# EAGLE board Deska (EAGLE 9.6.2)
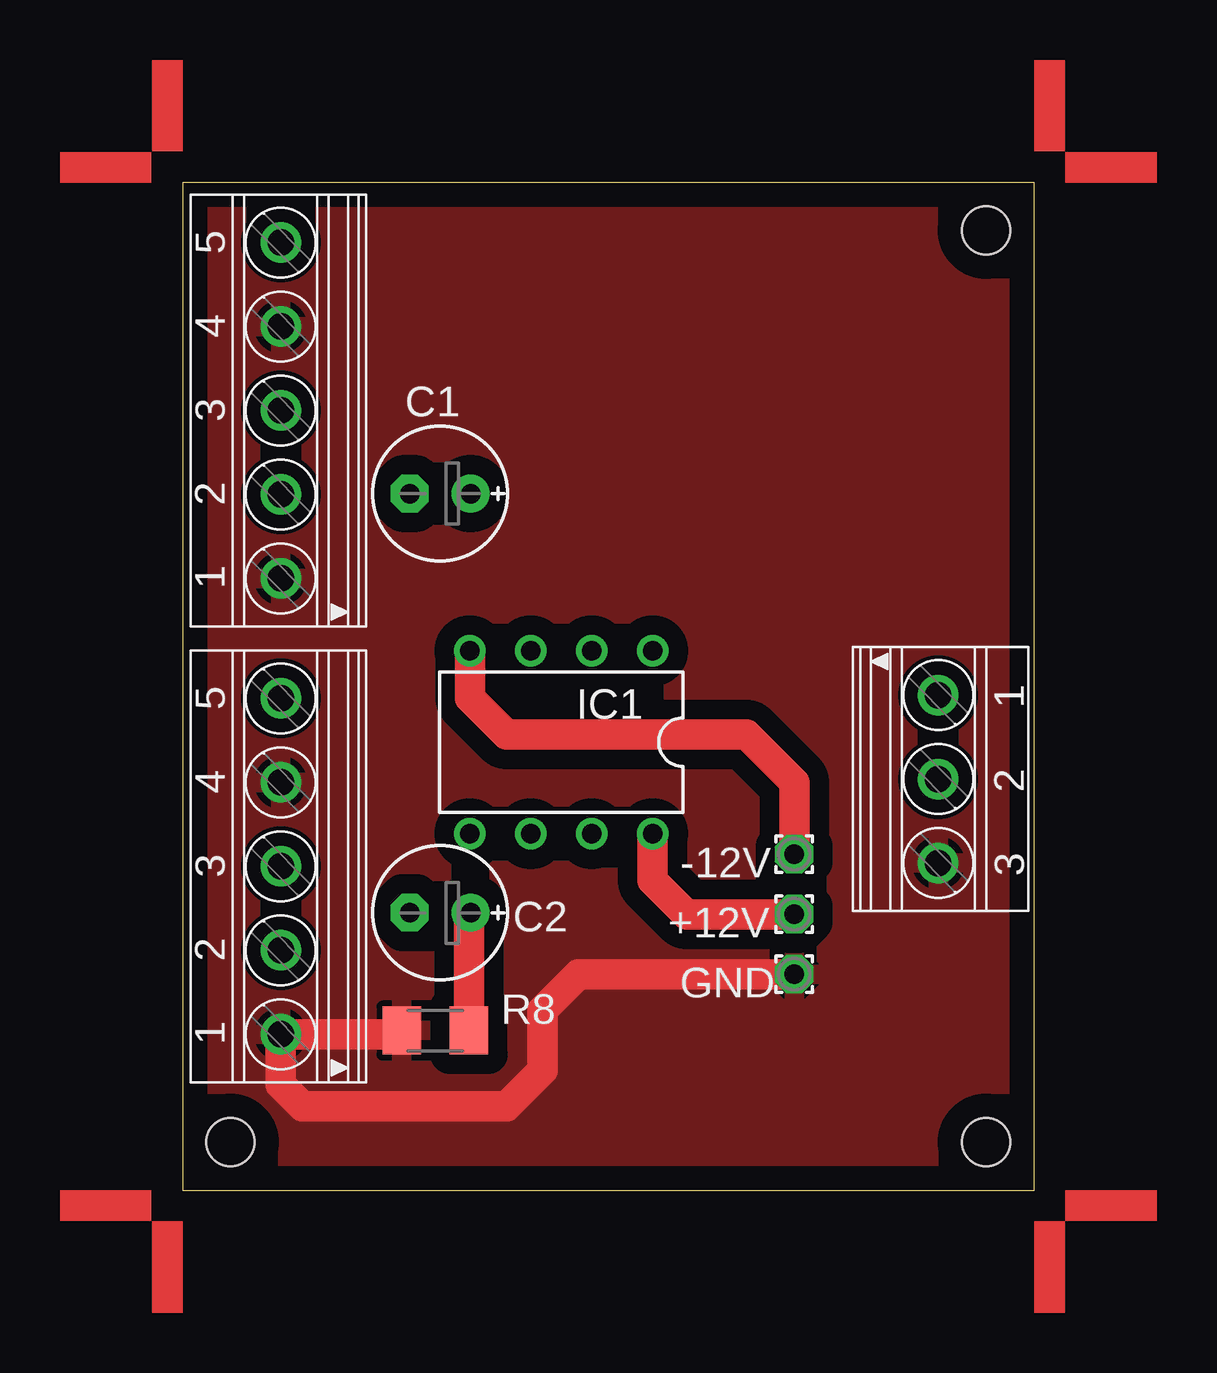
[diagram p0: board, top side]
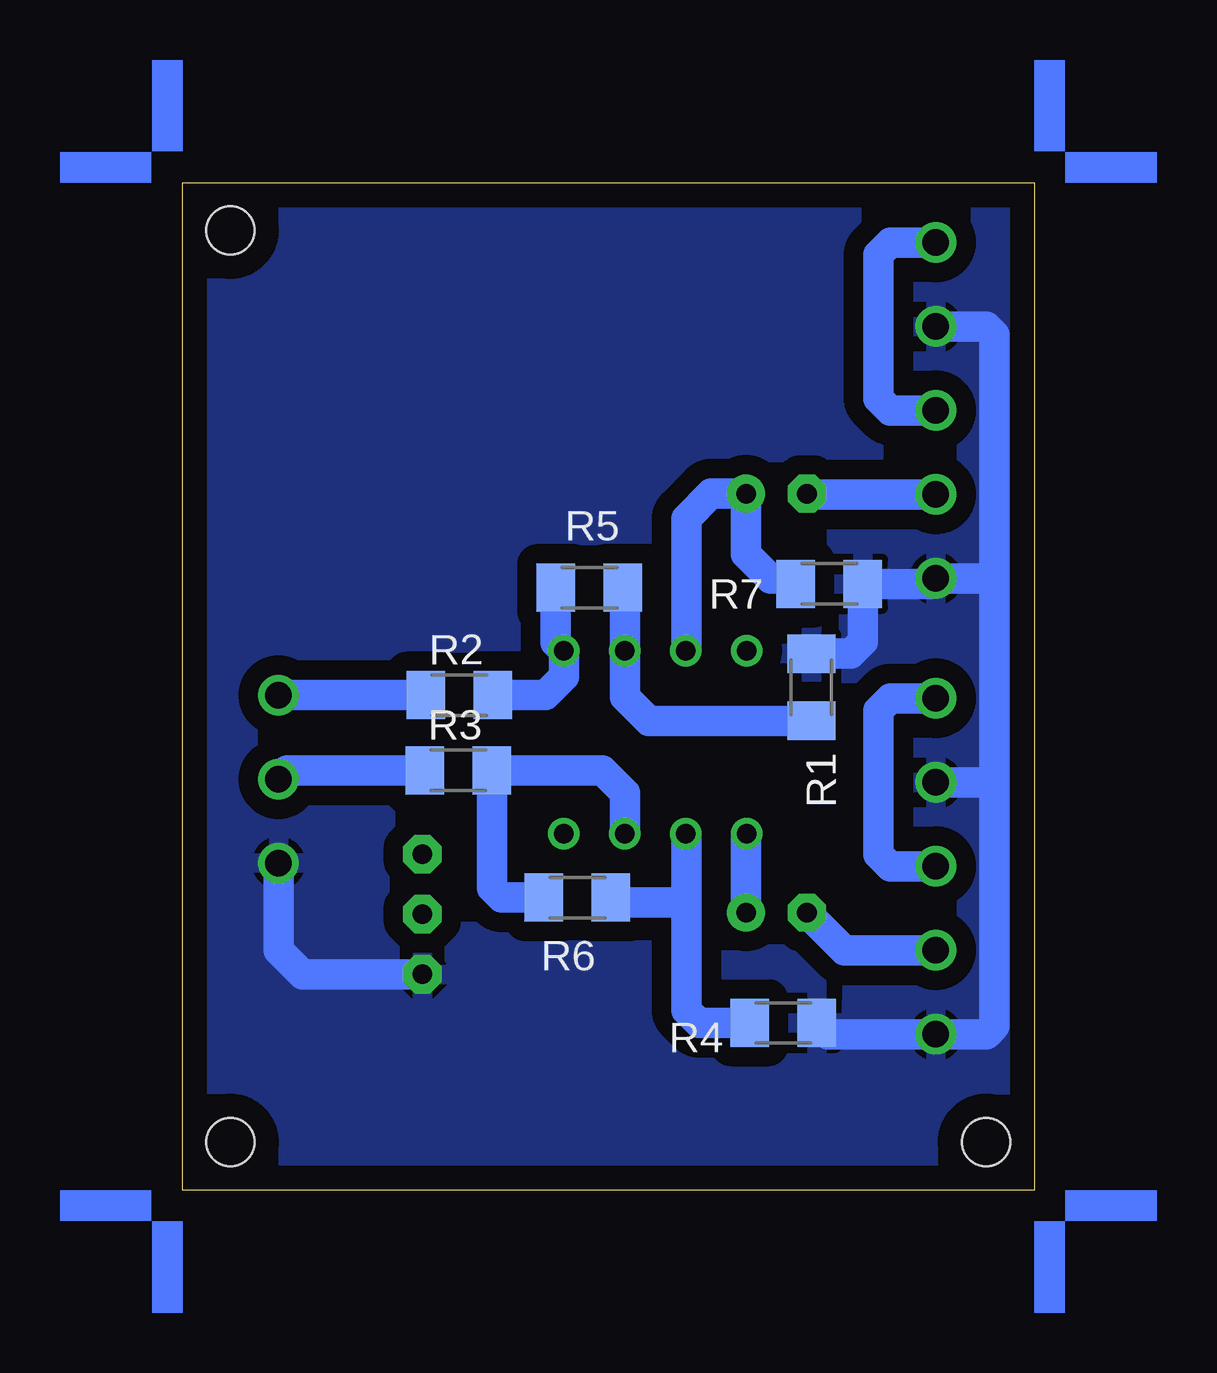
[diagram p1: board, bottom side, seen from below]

Size 35.5 x 42 mm. Coordinates in mm from the lower left corner, seen from the top.
Outline: 0,0 35.5,0 35.5,42 0,42 0,0
Copper layers (1*16): Top 0.035mm / dielectric 1.5mm / Bottom 0.035mm
Design rules "default": minimum track width 6mil, minimum drill 0.35mm, track to track 6mil, track to pad 6mil, pad to pad 6mil, via to via 6mil, smd to smd 6mil, copper to edge 40mil, drill to drill 6mil, minimum pad ring 10mil, minimum via ring 8mil, stop-mask expansion 4mil, vias tented up to drill 0mil, thermal gap 10mil
Holes 2 mm at 2,2 33.5,2 33.5,40

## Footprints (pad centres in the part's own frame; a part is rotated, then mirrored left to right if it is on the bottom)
1,6/0,8 = drill 0.813 pad 1.6 octagon: 1 0,0
E2,5-6E = drill 0.813 pad 1.575: + -1.27,0 | drill 0.813 pad 1.575 octagon: - 1.27,0
DIL08 = drill 0.813 pad 1.27: 1 -3.81,-3.81; 2 -1.27,-3.81; 3 1.27,-3.81; 4 3.81,-3.81; 5 3.81,3.81; 6 1.27,3.81; 7 -1.27,3.81; 8 -3.81,3.81
M1206 = smd 1.6 x 2: 1 -1.4,0; 2 1.4,0
1751277 = drill 1.1 pad 1.7: 1 -7,-0.1; 2 -3.5,-0.1; 3 0,-0.1; 4 3.5,-0.1; 5 7,-0.1
1751251 = drill 1.1 pad 1.7: 1 -3.5,-0.1; 2 0,-0.1; 3 3.5,-0.1

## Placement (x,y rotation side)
+12V  [1,6/0,8]  25.5,11.5 0 top
-12V  [1,6/0,8]  25.5,14 0 top
C1  2u2  [E2,5-6E]  10.74,29.03 180 top
C2  2u2  [E2,5-6E]  10.74,11.56 180 top
GND  [1,6/0,8]  25.5,9 0 top
IC1  TL072  [DIL08]  15.79,18.67 180 top
R1  [M1206]  9.29,20.96 270 bottom
R2  [M1206]  23.96,20.63 0 bottom
R3  [M1206]  24,17.5 0 bottom
R4  [M1206]  10.46,6.97 0 bottom
R5  [M1206]  18.54,25.11 180 bottom
R6  [M1206]  19.04,12.19 180 bottom
R7  [M1206]  8.54,25.27 180 bottom
R8  [M1206]  10.54,6.65 0 top
U$1  [ANGLE-SW1-16]  35.5,42 0 top
U$2  [ANGLE-SW1-16]  0,42 90 top
U$3  [ANGLE-SW1-16]  0,0 180 top
U$4  [ANGLE-SW1-16]  35.5,0 270 top
X1  [1751277]  4,32.5 90 top
X2  [1751277]  4,13.5 90 top
X4  [1751251]  31.6,17.13 270 top

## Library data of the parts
+12V -12V GND = wirepad
C1 C2 = rcl; SPICEPREFIX: C
IC1 = linear
R1-R8 = rcl; SPICEPREFIX: R
U$1-U$4 = marks
X1 X2 X4 = con-phoenix-350; OC_FARNELL: unknown; OC_NEWARK: unknown

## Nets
+12V: +12V.1 IC1.8
-12V: -12V.1 IC1.4
GND: GND.1 R1.1 R4.2 R7.1 R8.1 X1.1 X1.4 X2.1 X2.4 X4.3
N$1: C2.- X2.2
N$2: C1.- X1.2
N$3: C1.+ IC1.3 R7.2
N$4: C2.+ IC1.5 R8.2
N$5: IC1.2 R1.2 R5.1
N$6: IC1.1 R2.2 R5.2
N$7: IC1.7 R3.2 R6.2
N$8: IC1.6 R4.1 R6.1
N$9: R3.1 X4.2
N$10: R2.1 X4.1
N$11: X2.3 X2.5
N$12: X1.3 X1.5

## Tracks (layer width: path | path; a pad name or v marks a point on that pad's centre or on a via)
+12V
  Top 1.27: +12V.1 21,11.5 19.6,12.9 IC1.8
-12V
  Top 1.27: -12V.1 25.5,17 23.5,19 13.5,19 11.98,20.52 IC1.4
GND
  Top 1.27: R8.1 8.99,6.5 X2.1 4.1,4.4 5,3.5 13.5,3.5 15,5 15,7.5 16.5,9 GND.1
  Bottom 1.27: 1.65,17 1.65,6.85 2,6.5 X2.1 8.59,6.5 R4.2 | X1.4 2,36 1.65,35.65 1.65,25.5 | 1.65,25.5 1.65,17 | X2.4 1.65,17 | 1.65,25.5 X1.1 4.33,25.27 R7.1 7.14,22.86 7.64,22.36 R1.1 | GND.1 30.5,9 31.5,10 X4.3
  pour Top (isolate 0.813): 0,0 35.5,0 35.5,42 0,42
  pour Bottom (isolate 0.813): 0,0 35.5,0 35.5,42 0,42
N$1
  Bottom 1.27: C2.- 7.91,10 X2.2
N$2
  Bottom 1.27: C1.- 9.44,29 X1.2
N$3
  Bottom 1.27: IC1.3 14.5,22.5 14.5,28 13.47,29.03 C1.+ 12.01,26.51 11,25.5 10.17,25.5 R7.2
N$4
  Top 1.27: R8.2 11.94,11.49 C2.+
  Bottom 1.27: IC1.5 12.01,14.83 C2.+
N$5
  Bottom 1.27: R1.2 16.06,19.56 17.06,20.56 IC1.2 17.06,25.03 R5.1
N$6
  Bottom 1.27: R5.2 19.94,22.82 IC1.1 19.6,21.4 20.37,20.63 R2.2
N$7
  Bottom 1.27: IC1.7 17.06,16.56 18,17.5 R3.2 22.6,12.6 22.19,12.19 R6.2
N$8
  Bottom 1.27: IC1.6 14.5,14.84 14.5,12 | R4.1 13.97,6.97 14.5,7.5 14.5,12 | R6.1 17.45,12 14.5,12
N$9
  Bottom 1.27: X4.2 31.13,17.5 R3.1
N$10
  Bottom 1.27: R2.1 X4.1
N$11
  Bottom 1.27: X2.3 6,13.5 6.5,14 6.5,20 6,20.5 X2.5
N$12
  Bottom 1.27: X1.3 6,32.5 6.5,33 6.5,39 6,39.5 X1.5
